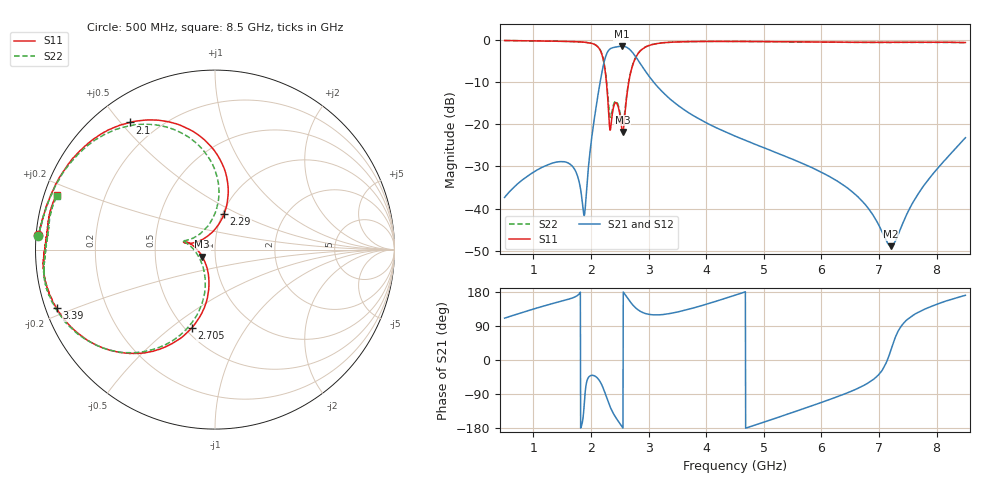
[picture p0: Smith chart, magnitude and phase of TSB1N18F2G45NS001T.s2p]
! TSB1N18F2G45NS001T  S-PARAMETER MODEL  ( General Type )
! Model Generated by TAIYO YUDEN Corporation (https://www.yuden.co.jp/en/)
! Version 2.0
! TAIYO YUDEN Control No. 080903
! Copyright(c) 2008 TAIYO YUDEN CO.,LTD. All Rights Reserved.
! Products Name : Multilayer Ceramic Devices
! Characteristics :
!  Passband freq : 2400-2500MHz ( At Passband , Insertion Loss : 2.3dB , VSWR 2.1 ),
!  Attenuation : 25dB min at 1710-1910MHz, 20dB min at 4800-5000MHz , Impedance : 50 Ohm ,
!  Case Size : 1.6 x 0.8 / 0.063 x 0.031 [mm/inch] , Thickness : 0.5 / 0.02 [mm/inch]
!  (Conditions: Temperature = 25 degC , DC Bias Current/Voltage = 0A / 0V)
! External Node Assignments :
!  1  o---|-------|---o  2
!  |  BPF  |
! GND o---|-------|---o GND
! Frequency Range : 500MHz  -  8.5GHz  [ 1601 STEP ]
# MHz S RI R 50
! Freq[MHz].  S11 Real  S11 Imag  S21 Real  S21 Imag  S12 Real  S12 Imag  S22 Real  S22 Imag
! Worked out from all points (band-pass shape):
!   1601 points, 500 MHz to 8.5 GHz, reference 50 ohm
!   highest |S21| = -1.47 dB at 2.53 GHz (marker M1); lowest = -48.9 dB at 7.205 GHz (marker M2)
!   |S21| within 3 dB of the highest: 2.242 GHz to 2.802 GHz (559.3 MHz wide, 22.2 % of centre)
!   lowest |S11| = -21.8 dB at 2.55 GHz (marker M3), VSWR 1.18, Z = 43.3 - j3.44 ohm
!   |S11| at or under -10 dB: 2.267 GHz to 2.655 GHz (387.8 MHz wide, 15.8 % of centre)
!   |S22| runs from -20.1 to -0.1 dB; largest |S21 - S12| = 0.002
!   S11 on the Smith chart (normalised r, x): 500 MHz: 0.01, +0.04; 2.1 GHz: 0.10, +0.53; 2.29 GHz: 1.02, +0.42; 2.705 GHz: 0.54, -0.59; 3.39 GHz: 0.03, -0.18; 8.5 GHz: 0.04, +0.17
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500  -0.9834 0.0803  -0.00474 0.0127  -0.00475 0.0128  -0.9844 0.0761
1490  -0.9203 0.2918  -0.0329 0.015  -0.0329 0.015  -0.9259 0.2709
1715  -0.8737 0.3884  -0.0284 0.00706  -0.0284 0.00704  -0.8861 0.362
1835  -0.8252 0.4642  -0.0142 -0.00157  -0.0142 -0.00157  -0.8443 0.4306
1900  -0.7865 0.5139  0.00118 -0.0101  0.00118 -0.0101  -0.8074 0.4794
2100  -0.4754 0.7085  0.1262 -0.1301  0.1262 -0.1303  -0.5266 0.6779
2215  -0.0224 0.5746  0.1268 -0.4876  0.1266 -0.4881  -0.0904 0.5804
2290  0.051 0.1989  -0.2147 -0.6947  -0.2141 -0.6958  0.00986 0.2319
2335  -0.0543 0.0659  -0.4465 -0.6496  -0.4465 -0.6505  -0.0737 0.096
2435  -0.1751 0.0441  -0.7357 -0.3766  -0.7362 -0.3777  -0.1815 0.0488
2530  -0.0935 -0.0072  -0.84 -0.0871  -0.8402 -0.0873  -0.1063 -0.0145
2550  -0.0708 -0.0395  -0.8439 -0.022  -0.8444 -0.0223  -0.0861 -0.0479
2705  -0.1308 -0.4372  -0.6275 0.3795  -0.6278 0.3795  -0.1526 -0.4357
3170  -0.8076 -0.425  -0.1325 0.2381  -0.1327 0.2382  -0.806 -0.4325
3390  -0.8816 -0.3266  -0.1071 0.1631  -0.1073 0.1634  -0.8795 -0.3434
4500  -0.9559 -0.1062  -0.0717 0.0114  -0.0717 0.0114  -0.9511 -0.1474
5835  -0.9464 0.0168  -0.0157 -0.0263  -0.0157 -0.0264  -0.9459 -0.0186
6675  -0.9358 0.087  0.00409 -0.0123  0.00408 -0.0123  -0.9343 0.0639
7170  -0.9301 0.1312  0.00367 0.000628  0.00368 0.000647  -0.9278 0.1136
7205  -0.9307 0.1364  0.00323 0.00155  0.00324 0.00154  -0.9255 0.12
7750  -0.9228 0.1929  -0.0115 0.0133  -0.0115 0.0133  -0.9191 0.1842
8500  -0.8829 0.303  -0.0684 0.0112  -0.0684 0.0112  -0.8798 0.2994
